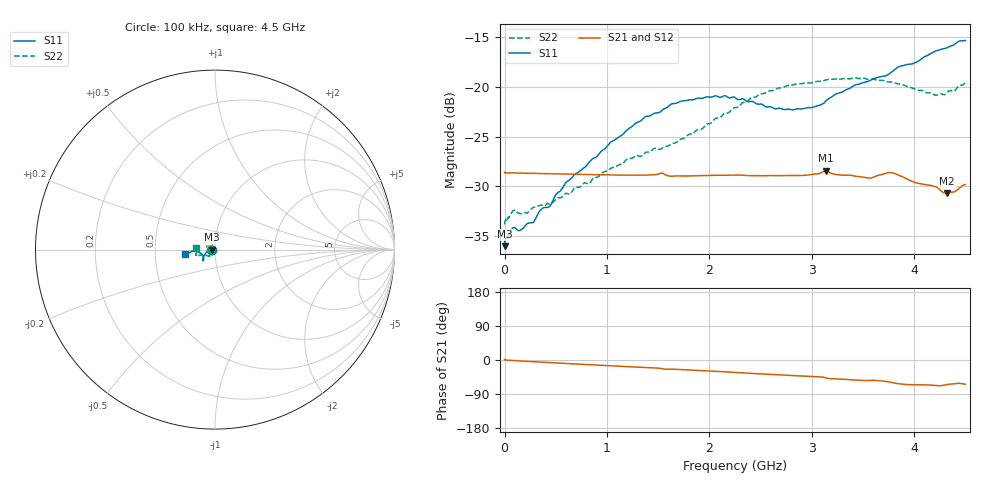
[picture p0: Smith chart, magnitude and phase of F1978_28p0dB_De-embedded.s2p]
! Integrated Device Technology
! Corporate Headquarters
! 6024 Silver Creek Valley Road
! San Jose, CA 95138  USA
! Phone:  1-408-284-8200
! Toll Free:  1-800-223-1366
! Webpage:  http://www.idt.com/
! Timing and RF Division
! 515 Groton Road, Suite 102
! Westford, MA 01886-6024
! Device:  F1978
! Description: 6-bit, 75 ohm, 0.5 dB Digital Step Attenuator
! Frequency:  5.0 MHz -  3.00 GHz
! Package:  4x4 mm QFN Plastic Package: 20 pin
! Ports:  2 RF, 11 DC
!  Pin  1  = D5 (16 dB)
!  Pin  2  = RF1  =  Port 1
!  Pin  3  = Serial Data In (DATA)
!  Pin  4  = Serial Clock (CLK)
!  Pin  5  = Serial Latch Enable (LE)
!  Pin  6  = VDD
!  Pin  7  = NC
!  Pin  8  = NC
!  Pin  9  = NC
!  Pin 10  = GND
!  Pin 11  = GND
!  Pin 12  = NC
!  Pin 13  = VMODE
!  Pin 14  = RF2  =  Port 2
!  Pin 15  = D4 (8 dB)
!  Pin 16  = D3 (4 dB)
!  Pin 17  = D2 (2 dB)
!  Pin 18  = NC
!  Pin 19  = D1 (1 dB)
!  Pin 20  = D0 (0.5 dB)
! State:  56
! Atten State:  28.0 dB
! Voltage:  +3.30 Volts
! Current:  0.595 mA
! Data:  The device was measured on a F1975 evaluation board which has
!  individual transmission lines to the RF pins.  Data was collected
!  using a calibrated network analyzer.  The evaluation board was
!  de-embedded using Automatic Fixture Removal (AFR).
!  The reference plane is the edge of the package pin.
! Misc:
!  Action Tracker AT0416
! Date Measured:  2018-02-08
! Date:  2018-03-26  MJV
! Note:
!  Integrated Device Technology supplies this data as a sample of measured
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# GHz S dB R 75
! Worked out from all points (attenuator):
!   291 points, 100 kHz to 4.5 GHz, reference 75 ohm
!   highest |S21| = -28.43 dB at 3.14 GHz (marker M1); lowest = -30.7 dB at 4.32 GHz (marker M2)
!   lowest |S11| = -36.0 dB at 100 kHz (marker M3), VSWR 1.03, Z = 72.7 - j0.0118 ohm
!   |S11| at or under -10 dB: start of sweep to end of sweep
!   |S22| runs from -33.8 to -19.1 dB; largest |S21 - S12| = 0.00018
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0.0001  -36.00 -179.7  -28.59 1.1  -28.59 1.2  -33.82 -178.8
0.011  -35.30 -178.1  -28.65 -0.3  -28.65 -0.3  -33.37 -176.7
0.08  -34.17 -176.6  -28.64 -1.3  -28.64 -1.3  -32.45 -169.6
0.14  -34.45 -175.9  -28.66 -2.3  -28.65 -2.3  -32.70 -161.2
0.22  -33.73 -179.7  -28.67 -3.6  -28.67 -3.6  -32.69 -155.1
0.28  -33.64 179.6  -28.69 -4.5  -28.69 -4.5  -32.11 -151.9
0.34  -32.50 178.1  -28.70 -5.4  -28.70 -5.4  -31.94 -146.9
0.44  -32.02 -179.7  -28.72 -6.8  -28.72 -6.8  -31.79 -138.7
0.6  -29.59 -176.2  -28.76 -9.2  -28.76 -9.1  -30.68 -132.9
0.76  -28.26 -169.5  -28.79 -11.4  -28.80 -11.4  -29.81 -128.9
1.28  -23.66 -153.2  -28.87 -18.5  -28.87 -18.5  -26.92 -124.6
1.52  -22.52 -145.9  -28.69 -21.9  -28.68 -21.9  -26.28 -131.2
1.88  -21.15 -138.9  -28.93 -27.1  -28.92 -27.1  -24.32 -147.0
2.26  -21.15 -137.3  -28.86 -32.9  -28.86 -32.9  -22.08 -157.9
2.64  -22.21 -147.6  -28.91 -38.5  -28.91 -38.5  -20.31 -159.3
3.02  -22.02 -164.2  -28.77 -43.8  -28.77 -43.8  -19.53 -159.9
3.14  -21.39 -167.0  -28.43 -47.3  -28.43 -47.3  -19.30 -160.4
3.56  -19.41 -177.3  -29.16 -54.1  -29.16 -54.1  -19.28 -165.8
3.76  -18.68 -175.9  -28.60 -58.3  -28.60 -58.3  -19.51 -169.5
4.2  -16.45 -172.7  -30.01 -67.0  -30.01 -67.0  -20.83 179.1
4.32  -16.08 -172.1  -30.70 -65.0  -30.69 -65.0  -20.62 176.7
4.5  -15.35 -171.8  -29.80 -64.1  -29.80 -64.1  -19.55 174.0
